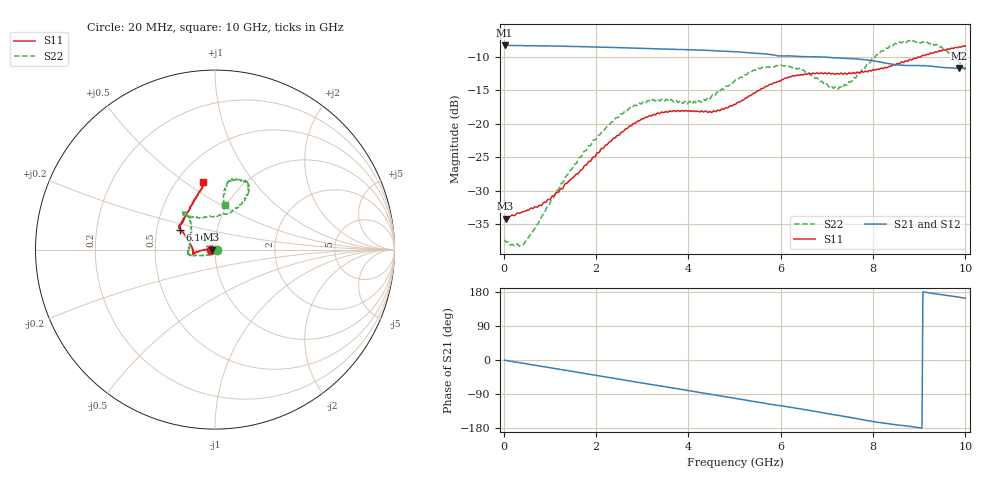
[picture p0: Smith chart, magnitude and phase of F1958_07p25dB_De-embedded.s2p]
! Integrated Device Technology
! Corporate Headquarters
! 6024 Silver Creek Valley Road
! San Jose, CA 95138  USA
! Phone:  1-408-284-8200
! Toll Free:  1-800-223-1366
! Webpage:  http://www.idt.com/
! Timing and RF Division
! 515 Groton Road, Suite 102
! Westford, MA 01886-6024
! Device:  F1958
! Description: 7-bit 0.25 dB Digital Step Attenuator
! Frequency:  0.001 -  6.000 GHz
! Package:  4x4 mm Thin QFN Plastic Package: 24 pin
! Ports:  2 RF, 12 DC
!  Pin  1  = D0
!  Pin  2  = VDD
!  Pin  3  = VMODE
!  Pin  4  = GND
!  Pin  5  = RF1  =  Port 1
!  Pin  6  = GND
!  Pin  7  = GND
!  Pin  8  = GND
!  Pin  9  = GND
!  Pin 10  = GND
!  Pin 11  = GND
!  Pin 12  = GND
!  Pin 13  = GND
!  Pin 14  = RF2  =  Port 2
!  Pin 15  = GND
!  Pin 16  = LE
!  Pin 17  = CLK
!  Pin 18  = DATA
!  Pin 19  = D6
!  Pin 20  = D5
!  Pin 21  = D4
!  Pin 22  = D3
!  Pin 23  = D2
!  Pin 24  = D1
! State:  29
! Atten State:  7.25 dB
! Voltage:  +3.30 Volts
! Current:  0.257 mA
! Data:  The device was measured on a F1958 evaluation board which has
!  individual transmission lines to the RF pins.  Data was collected
!  using a calibrated network analyzer.  The evaluation board was
!  de-embedded using Automatic Fixture Removal (AFR).
!  The reference plane is the edge of the package pin.
! Misc:
!  Action Tracker AT0419
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# GHz S dB R 50
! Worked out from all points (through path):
!   500 points, 20 MHz to 10 GHz, reference 50 ohm
!   highest |S21| = -8.23 dB at 20 MHz (marker M1); lowest = -11.7 dB at 9.86 GHz (marker M2)
!   group delay of S21, straight-line fit = 55.3 ps
!   lowest |S11| = -34.2 dB at 40 MHz (marker M3), VSWR 1.04, Z = 48.1 - j0.0789 ohm
!   |S11| at or under -10 dB: start of sweep to 8.976 GHz; 9.002581 GHz to 9.023046 GHz (20.46 MHz wide, 0.227 % of centre)
!   |S22| runs from -38.3 to -7.5 dB; largest |S21 - S12| = 0.0012
!   S11 on the Smith chart (normalised r, x): 20 MHz: 0.96, -0.00; 6.16 GHz: 0.66, +0.15; 10 GHz: 0.67, +0.59
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0.02  -34.14 -177.7  -8.23 -0.6  -8.23 -0.5  -37.34 -10.2
0.04  -34.20 -177.6  -8.24 -1.0  -8.24 -0.9  -37.62 -15.5
0.22  -33.73 178.1  -8.27 -4.7  -8.27 -4.6  -38.22 -35.8
0.44  -33.10 173.7  -8.29 -9.1  -8.29 -9.0  -37.94 -63.0
0.96  -31.29 174.9  -8.33 -19.6  -8.33 -19.5  -32.27 -109.8
1.7  -26.83 179.9  -8.44 -34.4  -8.43 -34.4  -24.65 -147.9
2.58  -21.20 -173.5  -8.61 -52.2  -8.59 -52.2  -18.47 -164.1
2.92  -19.56 -171.5  -8.68 -59.0  -8.67 -59.1  -16.93 -167.7
3.36  -18.43 -169.4  -8.78 -67.8  -8.78 -68.0  -16.48 -171.3
4.24  -18.22 -173.1  -8.95 -85.5  -8.96 -85.6  -16.56 159.2
5.02  -17.07 167.3  -9.20 -101.4  -9.21 -101.4  -13.44 131.1
5.54  -14.98 155.7  -9.46 -111.9  -9.47 -111.9  -11.70 128.5
6.16  -13.04 150.2  -9.82 -123.8  -9.83 -123.7  -11.46 131.2
6.68  -12.45 147.2  -9.95 -134.1  -9.97 -134.0  -12.72 126.4
7.06  -12.41 144.5  -10.05 -142.5  -10.06 -142.4  -14.44 108.1
7.3  -12.40 142.2  -10.14 -147.3  -10.15 -147.2  -14.45 90.4
7.9  -12.09 131.3  -10.45 -160.3  -10.45 -160.3  -10.91 61.8
8.34  -11.40 121.7  -10.98 -168.7  -10.99 -168.8  -8.57 59.7
8.76  -10.58 112.6  -11.27 -174.6  -11.28 -174.5  -7.56 65.1
9.26  -9.40 104.6  -11.38 176.3  -11.39 176.2  -7.89 75.8
9.86  -8.50 99.6  -11.68 165.8  -11.71 165.8  -10.71 79.5
10  -8.38 99.7  -11.66 162.8  -11.70 162.9  -11.95 77.5
